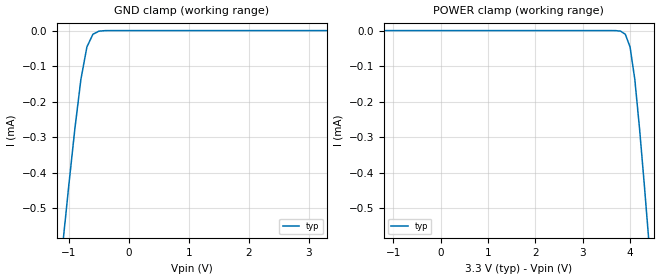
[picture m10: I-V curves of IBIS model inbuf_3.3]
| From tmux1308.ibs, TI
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| inbuf_3.3
[Model]   inbuf_3.3
Model_type   Input
Vinl = 0.8
Vinh = 1.15
|   typ   min   max
C_comp   4.014581e-14   NA   NA
[Voltage Range]   3.3   NA   NA
[Temperature Range]   27   NA   NA
[Power Clamp Reference]   3.3   NA   NA
[GND Clamp Reference]   0   NA   NA
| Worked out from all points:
|   GND clamp passes 1 mA (typ) near -1.33 V on its own axis
[GND Clamp]
|   Voltage   I(typ)   I(min)   I(max)
-6.6V     -10.7mA    NA         NA
-1.1V     -598uA     NA         NA
-1V       -432.7uA   NA         NA
-900mV    -275.6uA   NA         NA
-800mV    -137.3uA   NA         NA
-700mV    -46.04uA   NA         NA
-600mV    -10.45uA   NA         NA
-500mV    -1.642uA   NA         NA
-400mV    -165.4nA   NA         NA
3.3V      47.73pA    NA         NA
[POWER Clamp]
|   Voltage   I(typ)   I(min)   I(max)
-3.3V     3.404nA    NA         NA
3.8V      -1.642uA   NA         NA
3.9V      -10.45uA   NA         NA
4V        -46.04uA   NA         NA
4.1V      -137.3uA   NA         NA
4.2V      -275.6uA   NA         NA
4.3V      -432.7uA   NA         NA
4.4V      -598uA     NA         NA
6.6V      -4.566mA   NA         NA
